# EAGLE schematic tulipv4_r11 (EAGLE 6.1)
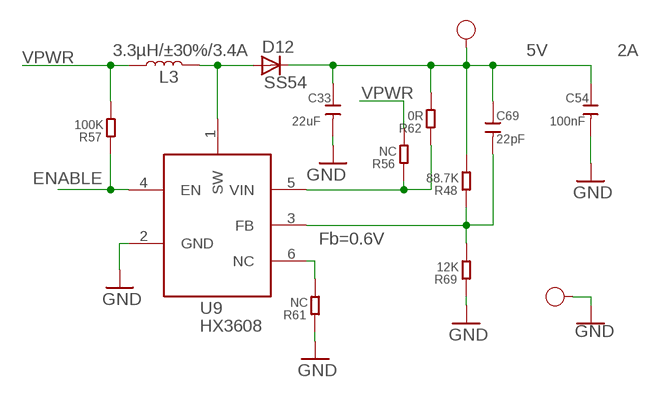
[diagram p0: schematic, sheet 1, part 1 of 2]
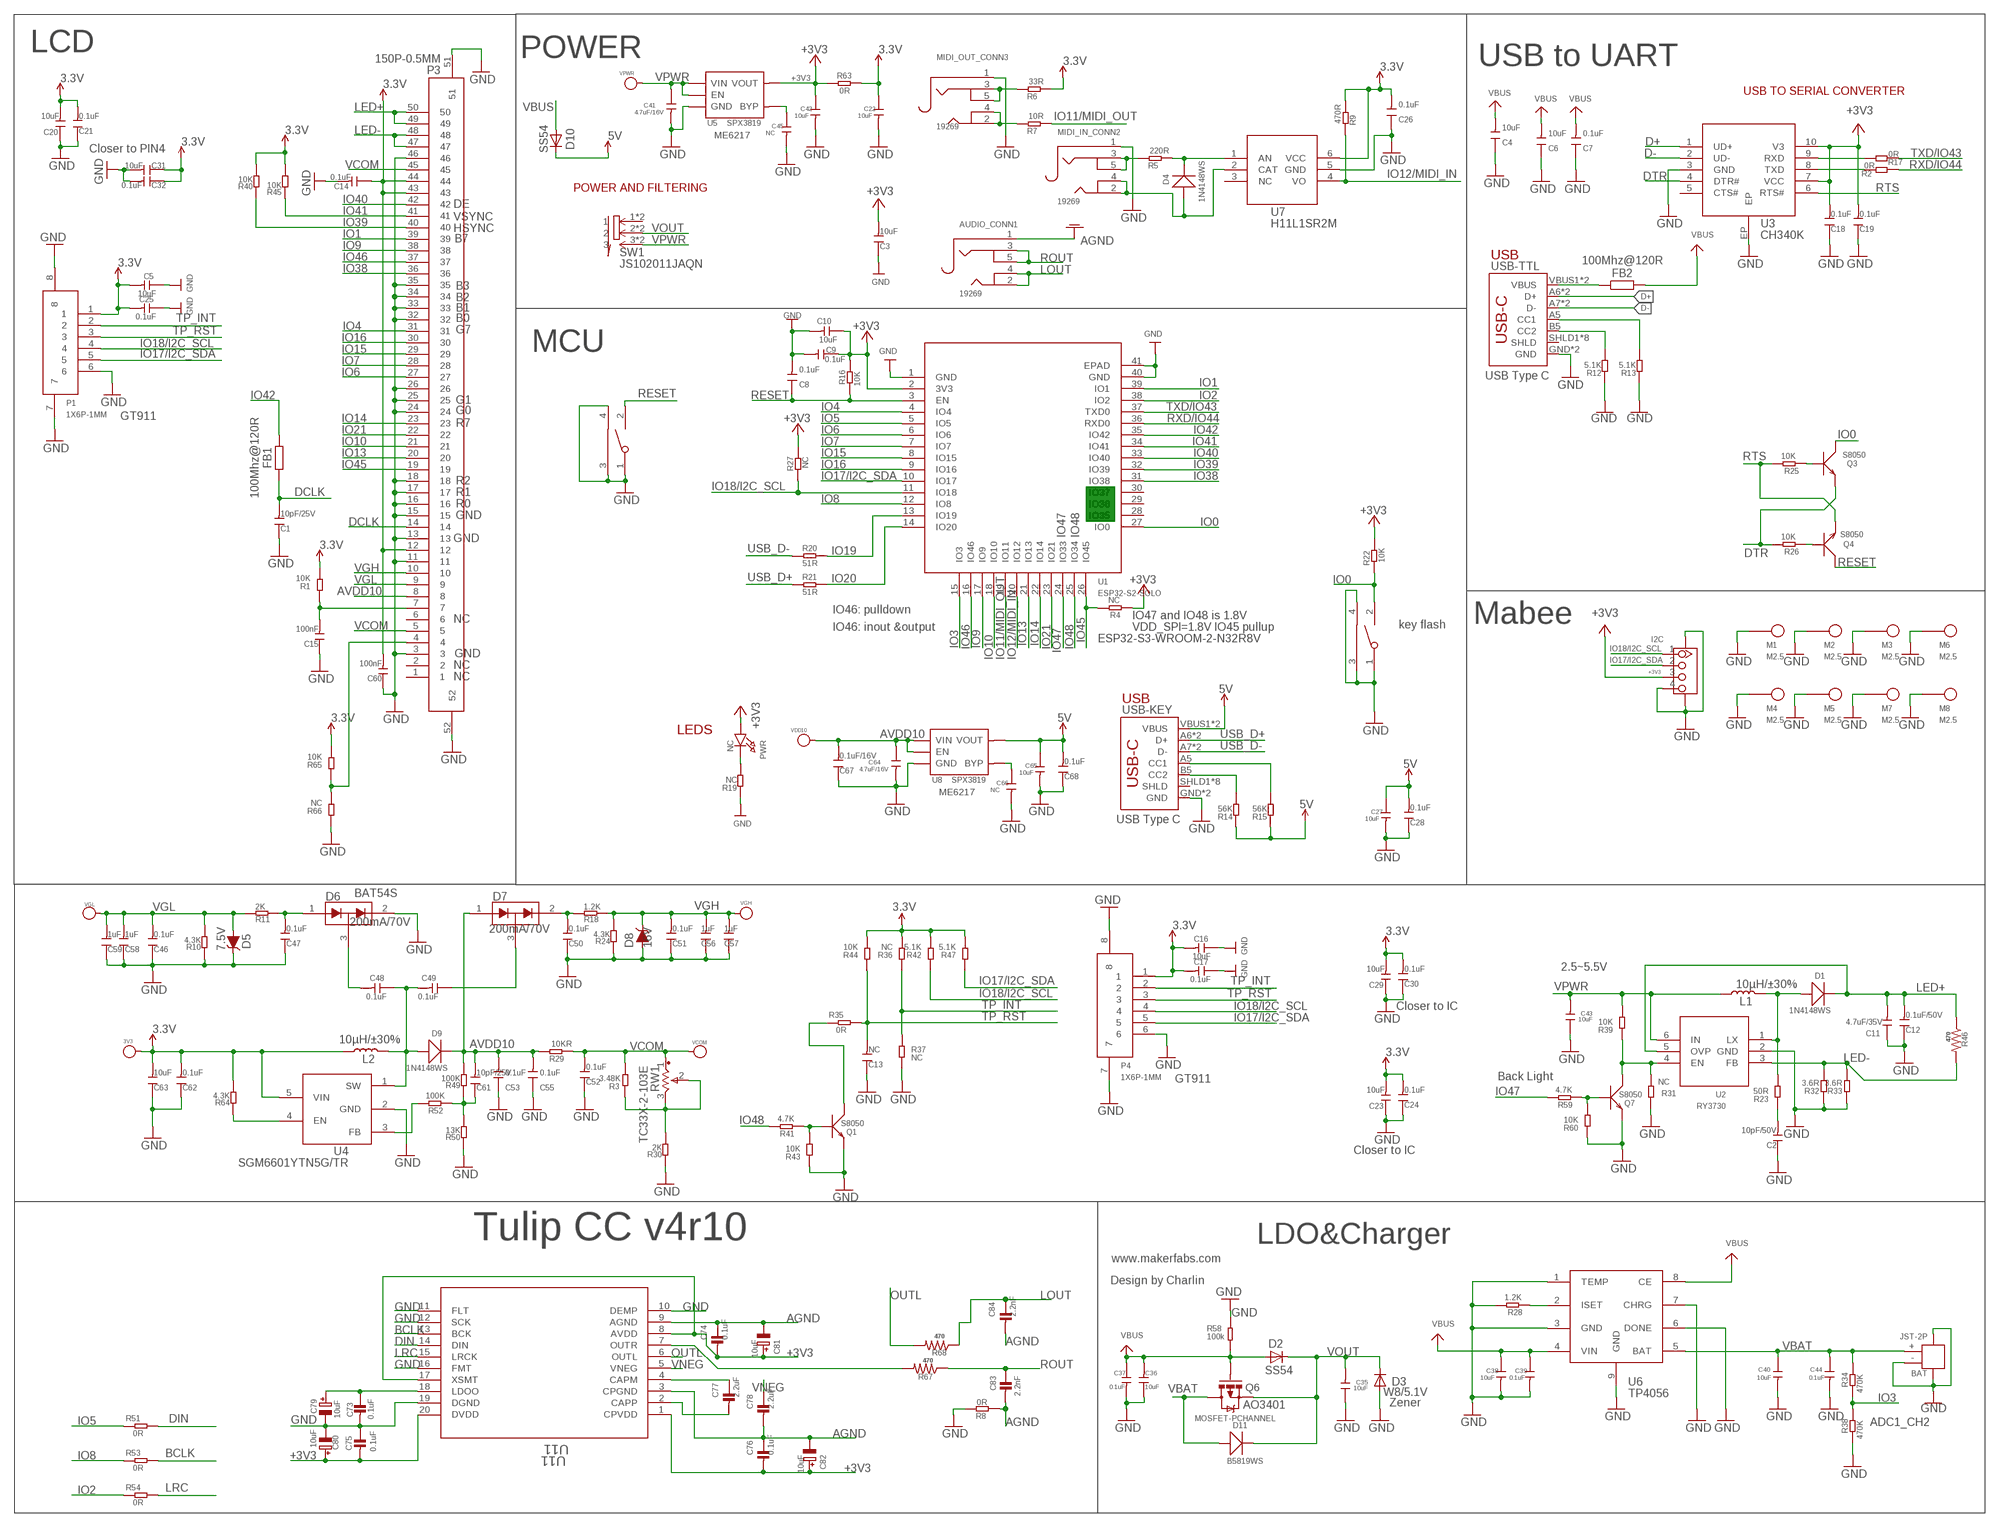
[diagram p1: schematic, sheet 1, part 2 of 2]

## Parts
3V3  PAD-TEST-POINT-CIRCLE'4545'  [TP_4545]
5V  TEST-POINT'4545'  [TP-D45MIL]
AUDIO_CONN1  19269  AUDIO_3.5MMJACK  [4UCONN_19269]
BAT  JST-2P  JST-2P-SMD'2.0'  [HW2-SMD-2.0-90D]
BOOT  TS24CA  [2*4*3.5MM]
C1  10pF/25V  DISCRETE_C-0603  [DISCRETE_C0603]
C2  10pF/50V  DISCRETE_C-0603  [DISCRETE_C0603]
C3  10uF  DISCRETE_C-0603  [DISCRETE_C0603]
C4  10uF  DISCRETE_C-0603  [DISCRETE_C0603]
C5  10uF  DISCRETE_C-0603  [DISCRETE_C0603]
C6  10uF  DISCRETE_C-0603  [DISCRETE_C0603]
C7  0.1uF  DISCRETE_C-0603  [DISCRETE_C0603]
C8  0.1uF  DISCRETE_C-0603  [DISCRETE_C0603]
C9  0.1uF  DISCRETE_C-0603  [DISCRETE_C0603]
C10  10uF  DISCRETE_C-0603  [DISCRETE_C0603]
C11  4.7uF/35V  DISCRETE_C-1206  [DISCRETE_C1206]
C12  0.1uF/50V  DISCRETE_C-0603  [DISCRETE_C0603]
C13  NC  DISCRETE_C-0603  [DISCRETE_C0603]
C14  0.1uF  DISCRETE_C-0603  [DISCRETE_C0603]
C15  100nF  DISCRETE_C-0603  [DISCRETE_C0603]
C16  10uF  DISCRETE_C-0603  [DISCRETE_C0603]
C17  0.1uF  DISCRETE_C-0603  [DISCRETE_C0603]
C18  0.1uF  DISCRETE_C-0603  [DISCRETE_C0603]
C19  0.1uF  DISCRETE_C-0603  [DISCRETE_C0603]
C20  10uF  DISCRETE_C-0603  [DISCRETE_C0603]
C21  0.1uF  DISCRETE_C-0603  [DISCRETE_C0603]
C22  10uF  C-0603  [0603]
C23  10uF  DISCRETE_C-0603  [DISCRETE_C0603]
C24  0.1uF  DISCRETE_C-0603  [DISCRETE_C0603]
C25  0.1uF  DISCRETE_C-0603  [DISCRETE_C0603]
C26  0.1uF  DISCRETE_C-0603  [DISCRETE_C0603]
C27  10uF  C-0603  [0603]
C28  0.1uF  DISCRETE_C-0603  [DISCRETE_C0603]
C29  10uF  DISCRETE_C-0603  [DISCRETE_C0603]
C30  0.1uF  DISCRETE_C-0603  [DISCRETE_C0603]
C31  10uF  DISCRETE_C-0603  [DISCRETE_C0603]
C32  0.1uF  DISCRETE_C-0603  [DISCRETE_C0603]
C33  22uF  CAP-0603  [C0603]
C35  10uF  C-0603  [0603]
C36  10uF  C-0603  [0603]
C37  0.1uF  C-0603  [0603]
C38  10uF  C-0603  [0603]
C39  0.1uF  C-0603  [0603]
C40  10uF  C-0603  [0603]
C41  4.7uF/16V  C-0603  [0603]
C42  10uF  C-0603  [0603]
C43  10uF  C-0603  [0603]
C44  0.1uF  C-0603  [0603]
C45  NC  C-0603  [0603]
C46  0.1uF  DISCRETE_C-0603  [DISCRETE_C0603]
C47  0.1uF  DISCRETE_C-0603  [DISCRETE_C0603]
C48  0.1uF  DISCRETE_C-0603  [DISCRETE_C0603]
C49  0.1uF  DISCRETE_C-0603  [DISCRETE_C0603]
C50  0.1uF  DISCRETE_C-0603  [DISCRETE_C0603]
C51  0.1uF  DISCRETE_C-0603  [DISCRETE_C0603]
C52  0.1uF  DISCRETE_C-0603  [DISCRETE_C0603]
C53  0.1uF  DISCRETE_C-0603  [DISCRETE_C0603]
C54  100nF  CAP-0603  [C0603]
C55  0.1uF  DISCRETE_C-0603  [DISCRETE_C0603]
C56  1uF  DISCRETE_C-0603  [DISCRETE_C0603]
C57  1uF  DISCRETE_C-0603  [DISCRETE_C0603]
C58  1uF  DISCRETE_C-0603  [DISCRETE_C0603]
C59  1uF  DISCRETE_C-0603  [DISCRETE_C0603]
C60  100nF  DISCRETE_C-0603  [DISCRETE_C0603]
C61  10pF/25V  DISCRETE_C-0603  [DISCRETE_C0603]
C62  0.1uF  DISCRETE_C-0603  [DISCRETE_C0603]
C63  10uF  DISCRETE_C-0603  [DISCRETE_C0603]
C64  4.7uF/16V  C-0603  [0603]
C65  10uF  C-0603  [0603]
C66  NC  C-0603  [0603]
C67  0.1uF/16V  DISCRETE_C-0603  [DISCRETE_C0603]
C68  0.1uF  DISCRETE_C-0603  [DISCRETE_C0603]
C69  22pF  CAP-0603  [C0603]
C73  0.1uF  CAP_CERAMIC0805-NOOUTLINE  [0805-NO@1]
C74  0.1uF  CAP_CERAMIC0805-NOOUTLINE  [0805-NO@1]
C75  0.1uF  CAP_CERAMIC0805-NOOUTLINE  [0805-NO@1]
C76  0.1uF  CAP_CERAMIC0805-NOOUTLINE  [0805-NO@1]
C77  2.2uF  CAP_CERAMIC0805-NOOUTLINE  [0805-NO@1]
C78  2.2uF  CAP_CERAMIC0805-NOOUTLINE  [0805-NO@1]
C79  10uF  CAP_ELECTROLYTICPANASONIC_C  [PANASONIC_C]
C80  10uF  CAP_ELECTROLYTICPANASONIC_C  [PANASONIC_C]
C81  10uF  CAP_ELECTROLYTICPANASONIC_C  [PANASONIC_C]
C82  10uF  CAP_ELECTROLYTICPANASONIC_C  [PANASONIC_C]
C83  2.2nF  CAP_CERAMIC0805-NOOUTLINE  [0805-NO@1]
C84  2.2nF  CAP_CERAMIC0805-NOOUTLINE  [0805-NO@1]
D1  1N4148WS  D'0805'  [SOD323]
D2  SS54  DIODE-DO-214AC  [DO-214AC]
D3  W8/5.1V  DIODE-SOD123  [SOD123]
D4  1N4148WS  D'0805'  [SOD323]
D5  7.5V  DIODE-ZENER-MMSZ5232BS  [SOD-323]
D6  200mA/70V  BAV99  [SOT23-3]
D7  200mA/70V  BAV99  [SOT23-3]
D8  16V  DIODE-ZENER-MMSZ5232BS  [SOD-323]
D9  1N4148WS  D'0805'  [SOD323]
D10  SS54  DIODE-DO-214AC  [DO-214AC]
D11  B5819WS  D'0805'  [SOD323]
D12  SS54  DIODE-DO-214AC  [DO-214AC]
FB1  100Mhz@120R  R-EU_R0805  [R0805]
FB2  100Mhz@120R  R-EU_R0805  [R0805]
GND  TEST-POINT'4545'  [TP-D45MIL]
I2C  GROVE-CONNECTOR-SMD'90D'  [HW4-SMD-2.0-90D]
L1  10µH/±30%  INDUCTOR-CR54-3.3UH  [CR54]
L2  10µH/±30%  INDUCTOR-CR54-3.3UH  [CR54]
L3  3.3µH/±30%/3.4A  INDUCTOR-CR54-3.3UH  [CR54]
M1  M2.5  [M2.5]
M2  M2.5  [M2.5]
M3  M2.5  [M2.5]
M4  M2.5  [M2.5]
M5  M2.5  [M2.5]
M6  M2.5  [M2.5]
M7  M2.5  [M2.5]
M8  M2.5  [M2.5]
MIDI_IN_CONN2  19269  AUDIO_3.5MMJACK  [4UCONN_19269]
MIDI_OUT_CONN3  19269  AUDIO_3.5MMJACK  [4UCONN_19269]
P1  1X6P-1MM  [1*6P-SMT1MM]
P3  150P-0.5MM  [1*50P-SMT0.5MM]
P4  1X6P-1MM  [1*6P-SMT1MM]
PWR  NC  LED0805_NOOUTLINE  [CHIPLED_0805_NOOUTLINE]
Q1  S8050  TRANSISTOR-NPN-SOT23  [SOT23]
Q3  S8050  TRANSISTOR-NPN-SOT23  [SOT23]
Q4  S8050  TRANSISTOR-NPN-SOT23  [SOT23]
Q6  MOSFET-PCHANNEL  [SOT23-3]
Q7  S8050  TRANSISTOR-NPN-SOT23  [SOT23]
R1  10K  DISCRETE_R-0603  [DISCRETE_R0603]
R2  0R  R-0603  [R0603]
R3  3.48K  DISCRETE_R-0603  [DISCRETE_R0603]
R4  NC  R-0603  [R0603]
R5  220R  R-0603  [R0603]
R6  33R  R-0603  [R0603]
R7  10R  R-0603  [R0603]
R8  0R  DISCRETE_R-0603  [DISCRETE_R0603]
R9  470R  R-0603  [R0603]
R10  4.3K  DISCRETE_R-0603  [DISCRETE_R0603]
R11  2K  DISCRETE_R-0603  [DISCRETE_R0603]
R12  5.1K  DISCRETE_R-0603  [DISCRETE_R0603]
R13  5.1K  DISCRETE_R-0603  [DISCRETE_R0603]
R14  56K  DISCRETE_R-0603  [DISCRETE_R0603]
R15  56K  DISCRETE_R-0603  [DISCRETE_R0603]
R16  10K  R-0603  [R0603]
R17  0R  R-0603  [R0603]
R18  1.2K  DISCRETE_R-0603  [DISCRETE_R0603]
R19  NC  DISCRETE_R-0603  [DISCRETE_R0603]
R20  51R  R-0603  [R0603]
R21  51R  R-0603  [R0603]
R22  10K  R-0603  [R0603]
R23  50R  DISCRETE_R-0603  [DISCRETE_R0603]
R24  4.3K  DISCRETE_R-0603  [DISCRETE_R0603]
R25  10K  R-0603  [R0603]
R26  10K  R-0603  [R0603]
R27  NC  R-0603  [R0603]
R28  1.2K  R-0603  [R0603]
R29  10KR  DISCRETE_R-0603  [DISCRETE_R0603]
R30  2K  DISCRETE_R-0603  [DISCRETE_R0603]
R31  NC  DISCRETE_R-0603  [DISCRETE_R0603]
R32  3.6R  DISCRETE_R-0603  [DISCRETE_R0603]
R33  3.6R  DISCRETE_R-0603  [DISCRETE_R0603]
R34  470K  R-0603  [R0603]
R35  0R  R-0603  [R0603]
R36  NC  DISCRETE_R-0603  [DISCRETE_R0603]
R37  NC  DISCRETE_R-0603  [DISCRETE_R0603]
R38  470K  R-0603  [R0603]
R39  10K  DISCRETE_R-0603  [DISCRETE_R0603]
R40  10K  DISCRETE_R-0603  [DISCRETE_R0603]
R41  4.7K  DISCRETE_R-0603  [DISCRETE_R0603]
R42  5.1K  DISCRETE_R-0603  [DISCRETE_R0603]
R43  10K  DISCRETE_R-0603  [DISCRETE_R0603]
R44  10K  DISCRETE_R-0603  [DISCRETE_R0603]
R45  10K  DISCRETE_R-0603  [DISCRETE_R0603]
R46  470  R-US_R0805  [R0805]
R47  5.1K  DISCRETE_R-0603  [DISCRETE_R0603]
R48  88.7K  DISCRETE_R-0603  [DISCRETE_R0603]
R49  100K  DISCRETE_R-0603  [DISCRETE_R0603]
R50  13K  DISCRETE_R-0603  [DISCRETE_R0603]
R51  0R  R-0603  [R0603]
R52  100K  DISCRETE_R-0603  [DISCRETE_R0603]
R53  0R  R-0603  [R0603]
R54  0R  R-0603  [R0603]
R56  NC  DISCRETE_R-0603  [DISCRETE_R0603]
R57  100K  DISCRETE_R-0603  [DISCRETE_R0603]
R58  100k  R-0603  [R0603]
R59  4.7K  DISCRETE_R-0603  [DISCRETE_R0603]
R60  10K  DISCRETE_R-0603  [DISCRETE_R0603]
R61  NC  DISCRETE_R-0603  [DISCRETE_R0603]
R62  0R  DISCRETE_R-0603  [DISCRETE_R0603]
R63  0R  R-0603  [R0603]
R64  4.3K  DISCRETE_R-0603  [DISCRETE_R0603]
R65  10K  DISCRETE_R-0603  [DISCRETE_R0603]
R66  NC  DISCRETE_R-0603  [DISCRETE_R0603]
R67  470  R-US_R0805  [R0805]
R68  470  R-US_R0805  [R0805]
R69  12K  DISCRETE_R-0603  [DISCRETE_R0603]
RST  TS24CA  [2*4*3.5MM]
RW1  TC33X-2-103E  [TC33-3MM-SMD]
SW1  JS102011JAQN  [SMD-6-2.5MM]
U1  ESP32­S2­SOLO  [ESP32-­S2-­SOLO]
U2  RY3730  [SOT23-6]
U3  CH340K  [ESOP-10-EP-150MIL]
U4  SGM6601YTN5G/TR  [SOT-23-5]
U5  SPX3819  [SOT23-5]
U6  TP4056  [SOP8-1.27P]
U7  H11L1SR2M  [SOP-6-2.54MM]
U8  SPX3819  [SOT23-5]
U9  HX3608  [SOT-23-6]
U11  U11  PCM5101APW  [PW20_TEX]
USB-KEY  USB_C5  [USB-C-16P-5]
USB-TTL  USB_C5  [USB-C-16P-5]
VCOM  PAD-TEST-POINT-CIRCLE'4545'  [TP_4545]
VDD10  PAD-TEST-POINT-CIRCLE'4545'  [TP_4545]
VGH  PAD-TEST-POINT-CIRCLE'4545'  [TP_4545]
VGL  PAD-TEST-POINT-CIRCLE'4545'  [TP_4545]
VPWR  PAD-TEST-POINT-CIRCLE'4545'  [TP_4545]

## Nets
3.3V: 3V3.T C5.2 C14.1 C16.2 C17.2 C20.2 C21.2 C22.1 C23.2 C24.2 C25.2 C26.2 C29.2 C30.2 C31.1 C32.1 C60.2 C62.2 C63.2 L2.P$1 P1.1 P3.12 P3.43 P3.44 P4.1 R1.2 R6.1 R9.1 R36.2 R40.2 R42.2 R44.2 R45.2 R47.2 R63.2 R64.2 R65.2 U4.5(VIN) U7.6(VCC)
5V: 5V.T C27.1 C28.2 C33.1 C54.1 C65.1 C68.2 C69.1 D10.C D12.C R14.1 R15.1 R48.2 R62.2 U8.5(VOUT) USB-KEY.VBUS1(VBUS) USB-KEY.VBUS2(VBUS)
+3V3: C3.2 C9.1 C10.1 C18.2 C19.2 C42.1 C74.2 C75.2 C76.2 C80.+ C81.+ C82.+ I2C.3 PWR.A R4.1 R16.2 R22.2 R27.2 R63.1 U1.2(3V3) U3.7(VCC) U3.10(V3) U5.5(VOUT) U11.1(CPVDD) U11.8(AVDD) U11.17(XSMT) U11.20(DVDD)
AGND: AUDIO_CONN1.1 C74.1 C76.1 C78.2 C81.- C82.- C83.2 C84.2 R8.1 U11.3(CPGND) U11.9(AGND)
AVDD10: C53.2 C55.2 C61.2 C64.1 C67.2 D7.1(A1) D9.- P3.8 R29.2 R49.2 U8.1(VIN) U8.3(EN) VDD10.T
BCLK: R53.2 U11.13(BCK)
D+: U3.1(UD+) USB-TTL.A6(D+) USB-TTL.B6(D+)
D-: U3.2(UD-) USB-TTL.A7(D-) USB-TTL.B7(D-)
DCLK: C1.2 FB1.1 P3.14
DIN: R51.2 U11.14(DIN)
DTR: Q3.2(E) R26.2 U3.4(DTR#)
ENABLE: R57.1 U9.4(EN)
GND: BAT.3 BAT.4 BAT.- BOOT.1 BOOT.3 BOOT.4 C1.1 C2.1 C3.1 C4.1 C5.1 C6.1 C7.1 C8.2 C9.2 C10.2 C11.1 C12.1 C13.1 C14.2 C15.1 C16.1 C17.1 C18.1 C19.1 C20.1 C21.1 C22.2 C23.1 C24.1 C25.1 C26.1 C27.2 C28.1 C29.1 C30.1 C31.2 C32.2 C33.2 C35.1 C36.1 C37.2 C38.2 C39.2 C40.2 C41.2 C42.2 C43.1 C44.2 C45.2 C46.1 C47.1 C50.1 C51.1 C52.1 C53.1 C54.2 C55.1 C56.1 C57.1 C58.1 C59.1 C60.1 C62.1 C63.1 C64.2 C65.2 C66.2 C67.1 C68.1 C73.2 C75.1 C79.- C80.- D3.A D5.C D6.2(C2) D8.A GND.T I2C.4 I2C.SS1 I2C.SS2 M1.1 M2.1 M3.1 M4.1 M5.1 M6.1 M7.1 M8.1 MIDI_IN_CONN2.1 MIDI_OUT_CONN3.1 P1.6 P1.7 P1.8 P3.3 P3.11 P3.13 P3.15 P3.16 P3.17 P3.18 P3.24 P3.25 P3.26 P3.32 P3.33 P3.34 P3.35 P3.46 P3.51 P3.52 P4.6 P4.7 P4.8 Q1.2(E) Q7.2(E) R8.2 R10.1 R12.1 R13.1 R19.1 R24.1 R28.2 R30.1 R31.1 R32.1 R33.1 R37.2 R38.1 R43.1 R50.1 R58.2 R60.1 R61.1 R66.1 R69.1 RST.1 RST.3 RST.4 U1.1(GND) U1.40(GND) U1.41(EPAD) U2.2(GND) U3.3(GND) U3.EP U4.2(GND) U5.2(GND) U6.1(TEMP) U6.3(GND) U6.6(DONE) U6.7(CHRG) U6.9(GND) U7.5(GND) U8.2(GND) U9.2(GND) U11.10(DEMP) U11.11(FLT) U11.12(SCK) U11.16(FMT) U11.19(DGND) USB-KEY.GND USB-KEY.GND2(GND) USB-TTL.GND USB-TTL.GND2(GND)
IO0: BOOT.2 Q3.3(C) R22.1 U1.27(IO0)
IO1: P3.39 U1.39(IO1)
IO2: R54.1 U1.38(IO2)
IO3: R34.1 R38.2 U1.15(IO3)
IO4: P3.31 U1.4(IO4)
IO5: R51.1 U1.5(IO5)
IO6: P3.27 U1.6(IO6)
IO7: P3.28 U1.7(IO7)
IO8: R53.1 U1.12(IO8)
IO9: P3.38 U1.17(IO9)
IO10: P3.21 U1.18(IO10)
IO11/MIDI_OUT: R7.1 U1.19(IO11)
IO12/MIDI_IN: R9.2 U1.20(IO12) U7.4(VO)
IO13: P3.20 U1.21(IO13)
IO14: P3.23 U1.22(IO14)
IO15: P3.29 U1.8(IO15)
IO16: P3.30 U1.9(IO16)
IO17/I2C_SDA: I2C.2 P1.5 P4.5 R47.1 U1.10(IO17)
IO18/I2C_SCL: I2C.1 P1.4 P4.4 R27.1 R42.1 U1.11(IO18)
IO19: R20.2 U1.13(IO19)
IO20: R21.2 U1.14(IO20)
IO21: P3.22 U1.23(IO21)
IO38: P3.36 U1.31(IO38)
IO39: P3.40 R40.1 U1.32(IO39)
IO40: P3.42 U1.33(IO40)
IO41: P3.41 R45.1 U1.34(IO41)
IO42: FB1.2 U1.35(IO42)
IO45: P3.19 R4.2 U1.26(IO45)
IO46: P3.37 U1.16(IO46)
IO47: R59.2 U1.24(IO33)
IO48: R41.2 U1.25(IO34)
LCD_RST: C15.2 P3.7 R1.1
LED+: C11.2 C12.2 D1.- P3.49 P3.50 R46.1 U2.5(OVP)
LED-: P3.47 P3.48 R32.2 R33.2 R46.2 U2.3(FB)
LOUT: AUDIO_CONN1.2 AUDIO_CONN1.4 C84.1 R68.1
LRC: R54.2 U11.15(LRCK)
N$1: C47.2 D6.1(A1) R11.1
N$2: Q4.1(B) R26.1
N$3: Q3.1(B) R25.1
N$4: C61.1 R49.1 R50.2 R52.1
N$5: P3.4 R65.1 R66.2
N$6: R15.2 USB-KEY.A5(CC1)
N$7: PWR.C R19.2
N$8: C48.2 D6.3(COM)
N$9: C48.1 C49.2 D9.+ L2.P$2 U4.1(SW)
N$10: R13.2 USB-TTL.A5(CC1)
N$11: R12.2 USB-TTL.B5(CC2)
N$12: C49.1 D7.3(COM)
N$13: C50.2 D7.2(C2) R18.2
N$14: R14.2 USB-KEY.B5(CC2)
N$15: R52.2 U4.3(FB)
N$16: R3.1 R30.2 RW1.2 RW1.3
N$17: D1.+ L1.P$2 R23.2 U2.1(LX)
N$18: Q1.3(C) R35.1
N$19: R64.1 U4.4(EN)
N$20: Q1.1(B) R41.1 R43.2
N$21: FB2.1 USB-TTL.VBUS1(VBUS) USB-TTL.VBUS2(VBUS)
N$22: C2.2 R23.1
N$23: MIDI_IN_CONN2.3 MIDI_IN_CONN2.5 R5.2
N$24: Q7.3(C) R31.2 R39.1 U2.4(EN)
N$25: D12.A L3.P$2 U9.1(SW)
N$26: D4.- R5.1 U7.1(AN)
N$27: MIDI_OUT_CONN3.3 MIDI_OUT_CONN3.5 R6.2
N$28: C69.2 R48.1 R69.2 U9.3(FB)
N$29: Q7.1(B) R59.1 R60.2
N$30: R28.1 U6.2(ISET)
N$31: R61.2 U9.6(NC)
N$32: R56.1 R62.1 U9.5(VIN)
N$33: C66.1 U8.4(BYP)
N$35: MIDI_OUT_CONN3.2 MIDI_OUT_CONN3.4 R7.2
N$36: D4.+ MIDI_IN_CONN2.2 MIDI_IN_CONN2.4 U7.2(CAT)
N$43: C73.1 C79.+ U11.18(LDOO)
N$44: R67.2 U11.7(OUTR)
N$45: C77.1 U11.4(CAPM)
N$46: R17.2 U3.9(RXD)
N$47: C77.2 U11.2(CAPP)
N$49: R2.2 U3.8(TXD)
N$76: C45.1 U5.4(BYP)
OUTL: R68.2 U11.6(OUTL)
RESET: C8.1 Q4.3(C) R16.1 RST.2 U1.3(EN)
ROUT: AUDIO_CONN1.3 AUDIO_CONN1.5 C83.1 R67.1
RTS: Q4.2(E) R25.2 U3.6(RTS#)
RXD/IO44: R2.1 U1.36(RXD0)
TP_INT: P1.2 P4.2 R36.1 R37.1
TP_RST: C13.2 P1.3 P4.3 R35.2 R44.1
TXD/IO43: R17.1 U1.37(TXD0)
USB_D+: R21.1 USB-KEY.A6(D+) USB-KEY.B6(D+)
USB_D-: R20.1 USB-KEY.A7(D-) USB-KEY.B7(D-)
VBAT: BAT.+ C40.1 C44.1 D11.+ Q6.3(D) R34.2 U6.5(BAT)
VBUS: C4.2 C6.2 C7.2 C36.2 C37.1 C38.1 C39.1 D2.A D10.A FB2.2 Q6.1(G) R58.1 U6.4(VIN) U6.8(CE)
VCOM: C52.2 P3.5 P3.45 R3.2 R29.1 RW1.1 VCOM.T
VGH: C51.2 C56.2 C57.2 D8.C P3.10 R18.1 R24.2 VGH.T
VGL: C46.2 C58.2 C59.2 D5.A P3.9 R10.2 R11.2 VGL.T
VNEG: C78.1 U11.5(VNEG)
VOUT: C35.2 D2.C D3.C D11.- Q6.2(S) SW1.2 SW1.2@1
VPWR: C41.1 C43.2 L1.P$1 L3.P$1 R39.2 R56.2 R57.2 SW1.3 SW1.3@1 U2.6(IN) U5.1(VIN) U5.3(EN) VPWR.T
Unconnected: P3.1 P3.2 P3.6 SW1.1 SW1.1@1 U1.28(IO35) U1.29(IO36) U1.30(IO37) U3.5(CTS#) U7.3(NC) USB-KEY.SHLD1(SHLD) USB-KEY.SHLD2(SHLD) USB-KEY.SHLD3(SHLD) USB-KEY.SHLD4(SHLD) USB-KEY.SHLD5(SHLD) USB-KEY.SHLD6(SHLD) USB-KEY.SHLD7(SHLD) USB-KEY.SHLD8(SHLD) USB-TTL.SHLD1(SHLD) USB-TTL.SHLD2(SHLD) USB-TTL.SHLD3(SHLD) USB-TTL.SHLD4(SHLD) USB-TTL.SHLD5(SHLD) USB-TTL.SHLD6(SHLD) USB-TTL.SHLD7(SHLD) USB-TTL.SHLD8(SHLD)

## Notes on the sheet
- LCD | POWER
- USB to UART
- USB TO SERIAL CONVERTER
- ME6217
- Closer to PIN4
- POWER AND FILTERING
- DE
- VSYNC
- HSYNC
- B7
- USB
- B3
- B2
- B1
- B0
- G7
- MCU
- USB Type C
- G1
- G0
- GT911
- R7
- R2
- R1
- R0
- GND
- IO47 | IO48
- GND
- IO46: pulldown
- IO47 and IO48 is 1.8V
- NC | Mabee
- IO46: inout &output | VDD_SPI=1.8V IO45 pullup | key flash
- ESP32-S3-WROOM-2-N32R8V
- GND
- NC
- NC
- USB
- LEDS
- ME6217
- USB Type C
- BAT54S
- 2A
- 2.5~5.5V
- Closer to IC
- Fb=0.6V
- GT911 | Back Light
- Closer to IC
- Tulip CC v4r10 | LDO&Charger
- www.makerfabs.com
- Design by Charlin
- AO3401 | Zener
- ADC1_CH2

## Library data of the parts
3V3 VCOM VDD10 VGH VGL VPWR = Discrete:PAD-TEST-POINT-CIRCLE; PARTNO: DNP
5V GND = Discrete-new:TEST-POINT; PARTNO: DNP
AUDIO_CONN1 MIDI_IN_CONN2 MIDI_OUT_CONN3 = microbuilder:AUDIO_3.5MMJACK: 3.5MM Audio Jack These are normally connected as follows, from left-to right on the schematic symbol above: Tip: Left Audio Inner Ring: Right Audio Shell: Common/GND
BAT = Connector-new:JST-2P-SMD: 2P-SMD-1.0-90D:320110054;2P-SMD-2.0-90D:320110026
BOOT RST = sale:TS24CA
C1-C21 C23-C26 C28-C32 C46-C53 C55-C63 C67 C68 = A9G:DISCRETE_C*: Ceramic Capacitors
C22 C27 C35-C45 C64-C66 = Discrete:C*: Ceramic Capacitors
C33 C54 C69 = Discrete-new:CAP: Ceramic Capacitors
C73-C78 C83 C84 = microbuilder:CAP_CERAMIC: Ceramic Capacitors
C79-C82 = microbuilder:CAP_ELECTROLYTIC: Electrolytic Capacitors
D1 D4 D9 D11 = Discrete:D*
D2 D3 D10 D12 = diode:DIODE-: DIODE
D5 D8 = SparkFun-DiscreteSemi:DIODE-ZENER: Zener Diode; PROD_ID: DIO-12442; VALUE: 5.6V
D6 D7 = SparkFun-DiscreteSemi:BAV99: Series-pair diode array Two small signal silicon diodes connected anode to cathode. Connections to all three nodes available. Link to datasheet SparkFun Products: SparkFun AutoDriver; PROD_ID: DIO-10647
FB1 FB2 = rcl:R-EU_: RESISTOR, European symbol
I2C = Connector-new:GROVE-CONNECTOR-SMD: 4P-SMD-2.0:320110030;4P-SMD-2.0-90D:320110032
L1 L2 = SparkFun-Coils:INDUCTOR: Inductors; PROD_ID: NDUC-11157; VALUE: 3.3µH/±30%/3.4A
L3 = SparkFun-Coils:INDUCTOR: Inductors; PROD_ID: NDUC-11157
M1-M8 = sale:M2.5
P1 P4 = sale:1X6P-1MM
P3 = sale:1*50P-0.5MM
PWR = microbuilder:LED: LED
Q1 Q3 Q4 Q7 = Discrete:TRANSISTOR-NPN*: NPN audion
Q6 = User-Submitted:MOSFET-PCHANNEL: Generic PMOSFET IRLML2244 - TRANS-11153 (SOT-23 -20V -4.3A) (1.Gate 2.Source 3.Drain) FQP27P06 - COM-10349 (TO-220 -60V -27A) (1.Gate 2.Source 3.Drain); PROD_ID: TRANS-08285
R1 R3 R8 R10-R15 R18 R19 R23 R24 R29-R33 R36 R37 R39-R45 R47-R50 R52 R56 R57 R59-R62 R64-R66 R69 = A9G:DISCRETE_R*
R2 R4-R7 R9 R16 R17 R20-R22 R25-R28 R34 R35 R38 R51 R53 R54 R58 R63 = Discrete:R*
R46 R67 R68 = adafruit:R-US_: RESISTOR, American symbol
RW1 = sale:TC33X-2-103E
SW1 = sale:JS102011JAQN
U1 = self:ESP32­S2­SOLO
U2 = sale:RY3730
U3 = sale:CH340K
U4 = sale:SGM6601YTN5G/TR
U5 U8 = IC:SPX3819
U6 = self:TP4056
U7 = sale:H11L1SR2M
U9 = self:HX3608
U11 = pcm5101apw:PCM5101APW; COPYRIGHT: Copyright (C) 2022 Ultra Librarian. All rights reserved.; DIGI-KEY_PART_NUMBER_1: PCM5101APW-ND; MANUFACTURER_PART_NUMBER: PCM5101APW; MFR_NAME: Texas Instruments
USB-KEY USB-TTL = USBC:USB_C: USB Type C 16Pin Connector Super Speed pins not available on the 16-pin purely SMD connector so this part is best for USB 2.0 implementations. D1 and D2 are tied together enabling D+/- no matter which way the cable is plugged into the connector. The two channel configuration pins (CC1/2) are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

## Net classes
0 default: width 0.203 mm, drill 0.305 mm, clearance 0.152 mm
1 vbat: width 0.254 mm, drill 0.305 mm, clearance 0.152 mm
